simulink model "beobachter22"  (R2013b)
settings: Solver=ode45  StartTime=0.0  StopTime=10.0  RelTol=1e-3
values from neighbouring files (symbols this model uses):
  A = [0 1 0 0 0 0    [beobachter_1.m]    (also in beobachter_2.m; beobachter_22.m; kalman_1.m = my_sys.a; kalman_10.m = my_sys.a)
  B = [0 1 0 0 0 0]'    [beobachter_1.m]    (also in beobachter_2.m; beobachter_22.m; kalman_1.m = my_sys.b; kalman_10.m = my_sys.b)
  C = [0 0 0 0 1 0]    [beobachter_1.m]    (also in beobachter_2.m; beobachter_22.m; kalman_1.m = my_sys.c; kalman_10.m = my_sys.c)
  D = 0    [aktiv_tilger_1.m]    (also in aktiv_tilger_12.m; aktiv_tilger_3.m = 2000; aktiv_tilger_31.m; beobachter_1.m)
  K = Kn(1:n)    [beobachter_2.m]    (also in beobachter_22.m; LQG_1.m = lqry(sys,10,1); LQR_1.m = Kn(1:6),      ki = -Kn(7),; pol_4.m)
  Ke = (place(A',C',p))'    [beobachter_1.m]    (also in beobachter_2.m; beobachter_22.m)
  ki = -Kn(n+1)    [beobachter_2.m]    (also in beobachter_22.m; kalman_12.m = -Kn(3); kalman_13.m = -Kn(4); kalman_d1.m = -Kn(4))
  Kr = 2000    [aktiv_tilger_2.m]    (also in beobachter_22.m = 5; fuellstnd_3.m = 10,; fuellstnd_31.m = 10,; kalman_12.m = Kn(1:2))
  smax = 0.05    [beobachter_22.m]    (also in PID_windup1.m = 0.3; pol_41.m = 0.02)
  x0 = [30,-20,0,0,0,0]    [beobachter_1.m]    (also in beobachter_2.m = [0,0,0,0,0.3,0]; beobachter_22.m = [0.1,0,0.1,0,0.3,0]; kalman_13.m = zeros(1,3); kalman_d1.m = zeros(1,3))

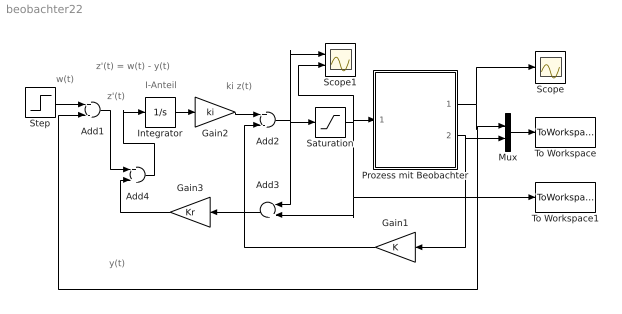
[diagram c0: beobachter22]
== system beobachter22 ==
  note: z'(t) = w(t) - y(t)
  note: y(t)
  note: w(t)
  note: ki z(t)
  note: z'(t)
  note: I-Anteil
  Add1 : Sum  Inputs=+-
  Add2 : Sum  Inputs=+-
  Add3 : Sum  Inputs=-+
  Add4 : Sum
  Gain1 : Gain  Gain=K  Multiplication=Matrix(K*u)
  Gain2 : Gain  Gain=ki
  Gain3 : Gain  Gain=Kr
  Integrator : Integrator
  Mux : Mux  Inputs=2
  Prozess mit Beobachter : Subsystem
  Saturation : Saturate  UpperLimit=smax  LowerLimit=-smax  LinearizeAsGain=off  ZeroCross=off
  Scope : Scope
  Scope1 : Scope  NumInputPorts=2
  Step : Step  SampleTime=0
  To Workspace : ToWorkspace  VariableName=yx  SampleTime=-1  SaveFormat=Structure With Time
  To Workspace1 : ToWorkspace  VariableName=us  SampleTime=-1  SaveFormat=Structure With Time
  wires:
  Step/1 -> Add1/1
  Integrator/1 -> Gain2/1
  Add2/1 -> Scope1/1, Saturation/1, Add3/1
  Gain1/1 -> Add2/2
  Prozess mit Beobachter/2(Geschätzter x(t)) -> Mux/2, Gain1/1
  Prozess mit Beobachter/1(Ausgang y(t)) -> Scope/1, Add1/2, Mux/1
  Mux/1 -> To Workspace/1
  Saturation/1 -> Add3/2, To Workspace1/1, Scope1/2, Prozess mit Beobachter/1(u(t))
  Add3/1 -> Gain3/1
  Gain2/1 -> Add2/1
  Add1/1 -> Add4/1
  Add4/1 -> Integrator/1
  Gain3/1 -> Add4/2

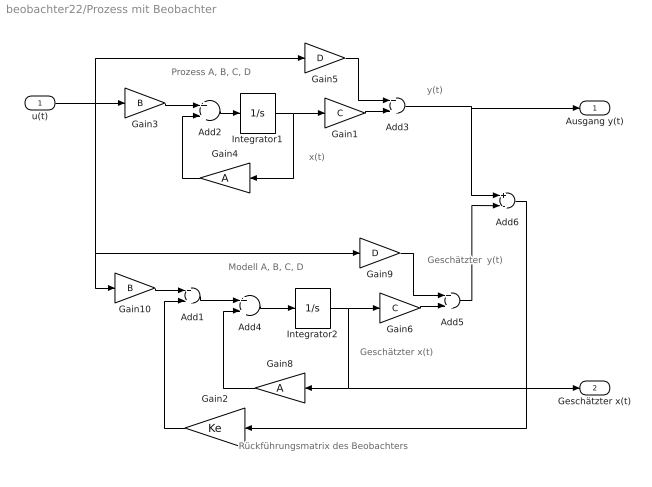
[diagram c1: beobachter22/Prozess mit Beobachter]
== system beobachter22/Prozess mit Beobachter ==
  note: Modell A, B, C, D
  note: Rückführungsmatrix des Beobachters
  note: Geschätzter x(t)
  note: y(t)
  note: Prozess A, B, C, D
  note: x(t)
  note: y(t)
  note: Geschätzter
  u(t) : Inport
  Add{1..5} (5 alike) : Sum
  Add6 : Sum  Inputs=+-
  Gain1 : Gain  Gain=C  Multiplication=Matrix(K*u)
  Gain10 : Gain  Gain=B  Multiplication=Matrix(K*u)
  Gain2 : Gain  Gain=Ke  Multiplication=Matrix(K*u)
  Gain3 : Gain  Gain=B  Multiplication=Matrix(K*u)
  Gain4 : Gain  Gain=A  Multiplication=Matrix(K*u)
  Gain5 : Gain  Gain=D  Multiplication=Matrix(K*u)
  Gain6 : Gain  Gain=C  Multiplication=Matrix(K*u)
  Gain8 : Gain  Gain=A  Multiplication=Matrix(K*u)
  Gain9 : Gain  Gain=D  Multiplication=Matrix(K*u)
  Integrator1 : Integrator  InitialCondition=x0
  Integrator2 : Integrator
  Ausgang y(t) : Outport
  Geschätzter x(t) : Outport  Port=2
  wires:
  Gain2/1 -> Add1/2
  Gain10/1 -> Add1/1
  Add4/1 -> Integrator2/1
  u(t)/1 -> Gain5/1, Gain3/1, Gain9/1, Gain10/1
  Integrator2/1 -> Gain6/1, Gain8/1, Geschätzter x(t)/1
  Gain9/1 -> Add5/1
  Gain4/1 -> Add2/2
  Gain3/1 -> Add2/1
  Add5/1 -> Add6/2
  Add6/1 -> Gain2/1
  Add2/1 -> Integrator1/1
  Gain1/1 -> Add3/2
  Gain5/1 -> Add3/1
  Add1/1 -> Add4/1
  Integrator1/1 -> Gain4/1, Gain1/1
  Add3/1 -> Add6/1, Ausgang y(t)/1
  Gain8/1 -> Add4/2
  Gain6/1 -> Add5/2
